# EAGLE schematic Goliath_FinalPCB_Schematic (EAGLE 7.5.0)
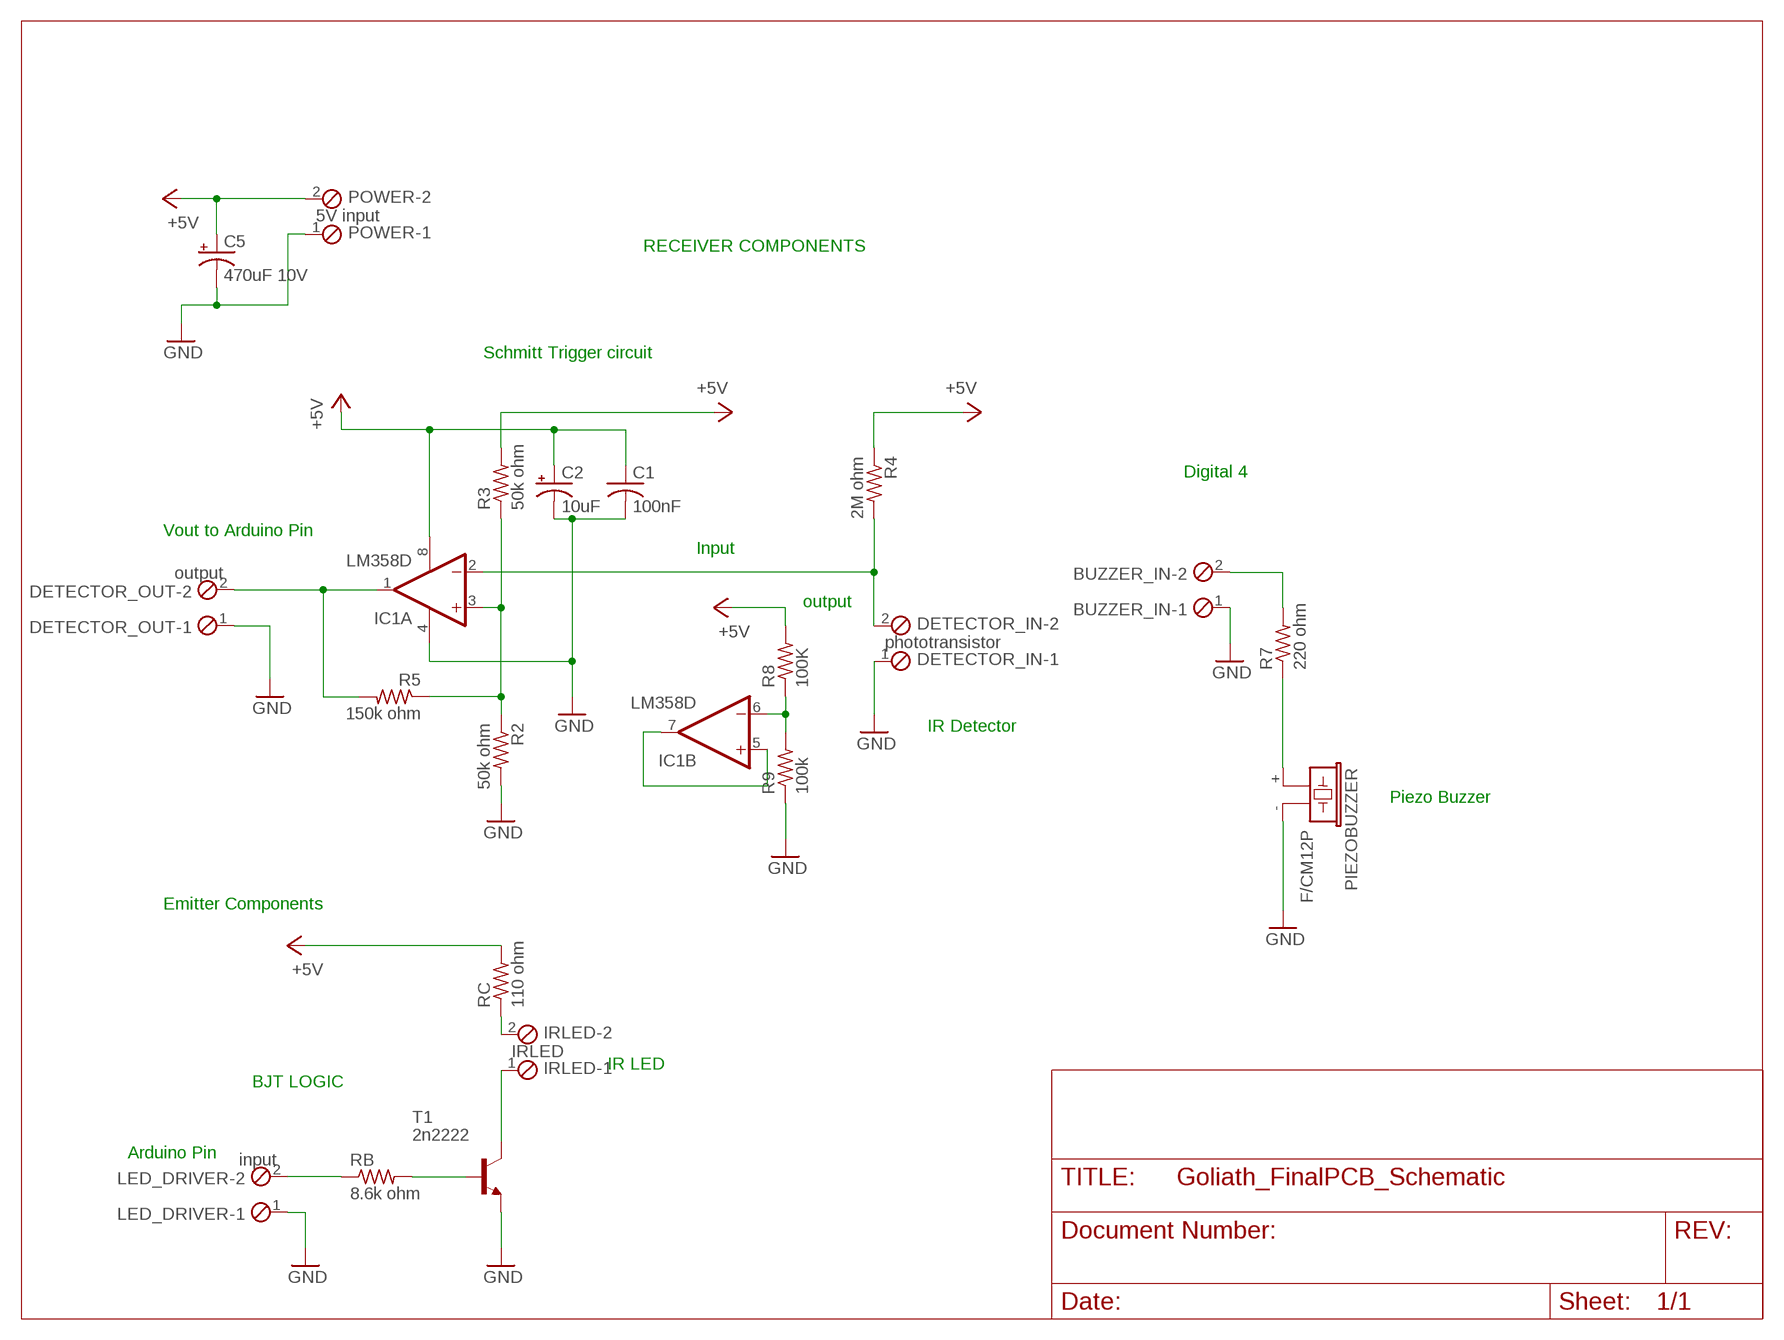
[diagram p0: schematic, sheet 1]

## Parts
BUZZER_IN  MPT2  [2POL254]
C1  100nF  C-USC0805  [C0805]
C2  10uF  CPOL-USE5-4  [E5-4]
C5  470uF 10V  CPOL-USE3.5-10  [E3,5-10]
DETECTOR_IN  phototransistor  MPT2  [2POL254]
DETECTOR_OUT  output  MPT2  [2POL254]
IC1  LM358D  [SO08]
IRLED  IRLED  MPT2  [2POL254]
LED_DRIVER  input  MPT2  [2POL254]
PIEZOBUZZER  F/CM12P  [F/CM12P]
POWER  5V input  MPT2  [2POL254]
R2  50k ohm  R-US_R0805  [R0805]
R3  50k ohm  R-US_R0805  [R0805]
R4  2M ohm  R-US_R0805  [R0805]
R5  150k ohm  R-US_R0805  [R0805]
R7  220 ohm  R-US_R1206  [R1206]
R8  100K  R-US_R0805  [R0805]
R9  100k  R-US_R0805  [R0805]
RB  8.6k ohm  R-US_R0805  [R0805]
RC  110 ohm  R-US_R1206  [R1206]
T1  2n2222  -NPN-SOT23-EBC  [SOT23-EBC]

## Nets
+5V: C1.1 C2.+ C5.+ IC1.8(P:V+) POWER.2 R3.2 R4.1 R8.2 RC.2
GND: BUZZER_IN.1 C1.2 C2.- C5.- DETECTOR_IN.1 DETECTOR_OUT.1 IC1.4(P:V-) LED_DRIVER.1 PIEZOBUZZER.- POWER.1 R2.2 R9.1 T1.E
N$1: DETECTOR_OUT.2 IC1.1(A:OUT) R5.2
N$2: PIEZOBUZZER.+ R7.1
N$3: DETECTOR_IN.2 IC1.2(A:-IN) R4.2
N$5: BUZZER_IN.2 R7.2
N$6: IC1.3(A:+IN) R2.1 R3.1 R5.1
N$7: IRLED.2 RC.1
N$10: IRLED.1 T1.C
N$11: RB.2 T1.B
N$12: LED_DRIVER.2 RB.1
N$14: IC1.5(B:+IN) IC1.7(B:OUT)
N$15: IC1.6(B:-IN) R8.1 R9.2

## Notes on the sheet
- RECEIVER COMPONENTS
- Schmitt Trigger circuit
- Digital 4
- Vout to Arduino Pin
- Input
- output
- IR Detector
- Piezo Buzzer
- Emitter Components
- IR LED
- BJT LOGIC
- Arduino Pin

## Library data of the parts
BUZZER_IN DETECTOR_IN DETECTOR_OUT IRLED LED_DRIVER POWER = con-phoenix-254:MPT2: PHOENIX CONNECTOR; OC_FARNELL: unknown; OC_NEWARK: unknown
C1 = rcl:C-US: CAPACITOR, American symbol
C2 C5 = rcl:CPOL-US: POLARIZED CAPACITOR, American symbol
IC1 = linear:LM358: OP AMP also LM158; LM258; LM2904 Source: http://cache.national.com/ds/LM/LM158.pdf
PIEZOBUZZER = buzzer:F/CM12P: BUZZER; OC_FARNELL: unknown; OC_NEWARK: unknown
R2-R5 R7-R9 RB RC = rcl:R-US_: RESISTOR, American symbol
T1 = transistor:*-NPN-: NPN Transistror BF959 corrected 2008.03.06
